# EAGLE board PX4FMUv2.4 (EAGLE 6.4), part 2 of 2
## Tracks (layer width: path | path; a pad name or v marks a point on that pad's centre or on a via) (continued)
GND  (via drill 0.2, 0.3) (continued)
  pour Top (isolate 0.254, rank 6, no thermals): 60.35,19.71 60.35,15.85 59.74,15.24 59.74,11.07 59.94,10.87 61.57,10.87 61.67,10.97 61.67,19.71 61.47,19.91 60.55,19.91
  pour Top (isolate 0.254, rank 6, no thermals): 51.71,35.36 59.03,35.26 59.13,35.15 59.13,28.85 59.03,28.75 51.71,28.85 51.51,29.06 51.61,35.26
  pour Top (isolate 0.254, rank 6, no thermals): 28.24,36.47 37.08,36.47 37.49,36.88 37.49,40.44 28.14,40.44 28.04,36.68
  pour Top (isolate 0.254, rank 6, no thermals): 52.22,17.88 57,17.88 57,13.31 52.22,13.31
  pour Top (isolate 0.254, rank 6, no thermals): 67.26,16.66 67.87,16.66 68.17,16.97 68.17,17.58 68.48,17.88 69.49,17.88 69.7,17.68 69.7,15.75 69.49,15.54 67.16,15.54 67.06,15.65 67.06,16.56 67.16,16.66
GPIO_EXT_1  (via drill 0.2)
  Top 0.152: v33.63,15.85 33.53,15.85 32.41,16.97 31.72,16.97 U101.8
  Vertical 0.152: v33.63,15.85 34.85,17.07 34.85,30.18 35.76,31.09 v38,31.09
  Bottom 0.152: J403.6 47.39,30.42 46.13,29.16 40.03,29.16 38.1,31.09 v38,31.09
GYRO_DRDY  (via drill 0.2)
  Top 0.152: U501.6 62.9,13.11 62.48,13.11 v61.98,12.6 | v43.48,12.29 43.48,12.5 42.8,13.18 U101.35 | U502.6 57.6,8.32 v57.81,8.33 | X503.5 57.13,4.6 v58.22,5.69
  Horizontal 0.152: v43.48,12.29 43.48,11.48 43.89,11.07 52.02,11.07 v52.22,11.28 | v53.14,5.69 v58.22,5.69
  Vertical 0.152: v58.22,5.69 58.22,8.13 58.01,8.33 v57.81,8.33 57.51,8.64 57.51,10.57 57.3,10.77 57.3,10.97 57.71,11.38 58.12,11.38 58.73,10.77 61.57,10.77 61.98,11.18 v61.98,12.6 | v52.22,11.28 52.22,6.6 v53.14,5.69
IO-!RESET  (via drill 0.2)
  Top 0.152: v19.51,16.66 19.51,16.71 U801.7 | U1002.3 13.66,7.26 v13.61,7.21 | v24.38,5.99 C801.P$2 23.77,4.77 23.77,3.09 S801.A1
  Horizontal 0.152: v13.61,7.21 14.94,8.53 v20.52,8.53
  Vertical 0.152: v20.52,8.53 20.52,15.65 v19.51,16.66
  Bottom 0.152: v24.38,5.99 22.86,5.99 20.52,8.33 v20.52,8.53
IO-!VDD_SERVO_IN_FAULT  (via drill 0.2)
  Top 0.152: U1001.4 12.46,4.74 v12.19,4.47 | v25.91,14.73 25.91,15.41 U801.38
  Horizontal 0.152: v12.19,4.47 12.39,4.27 15.65,4.27 16.46,5.08 16.46,7.21 17.27,8.03 20.73,8.03 21.03,8.33 22.15,8.33 25.7,11.89 25.7,13.51 25.6,13.61 25.6,14.43 v25.91,14.73
IO-BOOT0  (via drill 0.2)
  Top 0.152: U801.44 25.26,19.01 | 25.26,19.01 R801.P$1 | 25.26,19.01 25.26,19.14 23.67,20.73 v23.16,20.73
  Bottom 0.152: v23.16,20.73 23.57,20.73 IO-BOOT1101.P$1
IO-BOOT1
  Top 0.152: R802.P$1 17.92,9.54 U801.20
IO-CH1
  Top 0.152: U801.10 17.03,17.07 15.85,17.07 15.57,16.79 U902.9
IO-CH1-PROT
  Top 0.406: J901.28 8.33,21.97 8.33,19.21 R917.P$2
IO-CH2
  Top 0.152: U801.11 16.73,16.66 16.26,16.66 15.88,16.29 U902.8
IO-CH3
  Top 0.152: U902.7 16.22,15.79 16.87,15.14 22.05,15.14 23.57,16.66 23.57,18.02 U801.45
IO-CH4  (via drill 0.2)
  Top 0.152: U902.6 15.5,15.29 v15.54,15.24 | v22.96,18.12 U801.46
  Horizontal 0.152: v22.96,18.12 22.49,18.12 19.61,15.24 v15.54,15.24
IO-CH5
  Top 0.152: U902.5 15.49,14.79 16.05,14.22 16.05,11.68 16.26,11.48 17.03,11.48 U801.16
IO-CH6
  Top 0.152: U902.4 15.38,14.29 15.75,13.92 15.75,11.48 16.05,11.18 17.43,11.18 U801.17
IO-CH7
  Top 0.152: U902.3 15.27,13.79 15.44,13.61 15.44,11.28 15.85,10.87 17.83,10.87 U801.18
IO-CH8
  Top 0.152: U801.19 18.23,10.57 15.65,10.57 15.14,11.07 15.14,12.09 15.04,12.19 14.02,12.19 13.76,12.46 U902.1
IO-CH8-PROT
  Top 0.152: 8.44,10.47 R905.P$2
  Top 0.406: J901.7 7.72,7.64 7.72,9.75 8.44,10.47
IO-SWCLK  (via drill 0.2)
  Top 0.152: U801.37 26.44,15.24 v26.42,15.24
  Bottom 0.152: JX802.4 16.1,18.85 17.37,17.58 23.06,17.58 25.4,15.24 v26.42,15.24
IO-SWDIO  (via drill 0.2)
  Top 0.152: v25.09,14.02 25.09,13.96 U801.34
  Bottom 0.152: JX802.2 15.75,17.58 16.15,17.17 22.66,17.17 25.09,14.73 v25.09,14.02
IO-SWO  (via drill 0.2)
  Top 0.152: U801.39 25.74,15.95 v25.7,15.95
  Bottom 0.152: JX802.6 22.15,20.12 25.7,16.56 v25.7,15.95
IO-USART1_RX  (via drill 0.2)
  Top 0.152: U801.31 v24.69,12.24
  Horizontal 0.152: v24.69,12.24 24.13,12.8 15.44,12.8 14.83,13.41 v13.01,13.41 | v11.68,0.61 18.95,0.61 v19.1,0.46
  Vertical 0.152: v15.75,27.13 13.01,24.38 v13.01,13.41 13.01,10.16 11.38,8.53 11.38,2.85 11.68,2.54 v11.68,0.61
  Bottom 0.152: J801.P$3 15.93,27.31 v15.75,27.13 | v19.1,0.46 19.25,0.61 19.71,0.61 JX801.2
IO-USART1_TX  (via drill 0.2)
  Top 0.152: v24.08,23.06 24.18,23.16 R101.P$2 | v24.08,12.19 24.08,12.14 U801.30
  Vertical 0.152: v24.08,23.06 v24.08,12.19 23.27,12.19 22.86,11.79 22.86,11.18 23.27,10.77 23.27,3.45 22.25,2.44 v22.15,2.44
  Bottom 0.152: JX801.1 22.86,2.13 22.55,2.44 v22.15,2.44
IO-VDD_3V3  (via drill 0.2, 0.3)
  Top 0.254: U801.48 22.45,20.49 C803.P$1 22.45,21.45 v22.35,21.54 21.95,21.95 D701.C | C804.P$1 27.32,14.13 v27.23,14.22 27.23,13.55 U801.36 | v11.28,12.8 11.26,12.82 U902.19 | v14.73,12.7 14.73,13.26 U902.2 | v13.82,16.26 13.76,16.32 U902.10 13.94,17.48 14.22,17.48 | U801.9 17.33,17.48 14.22,17.48 | C802.P$1 21.45,9.25 v21.54,9.35 21.38,9.5 U801.24 | C903.P$1 14.32,17.57 14.22,17.48 | U903.8 13.15,3.72 C901.P$1 12.61,3.76 v12.29,3.76
  Bottom 0.406: J702.1 22.32,21.57 v22.35,21.54 | JX802.1 11.48,17.58 v12.19,18.29
  other vias: 11.07,10.36 11.58,10.36
  pour Power: 7.72,23.98 7.72,0 28.04,0 28.04,16.66 20.73,23.98
  pour Top (isolate 0.254, rank 3, no thermals): 13.31,9.14 13.31,10.36 13.21,10.46 12.29,10.46 11.89,10.87 11.89,11.58 11.79,11.68 10.97,11.68 10.87,11.58 10.87,9.55 10.97,9.45 11.89,9.45 12.29,9.86 12.9,9.86 13,9.75 13,9.14 13.11,9.04 13.21,9.04
IO-VDD_5V5  (via drill 0.3)
  Top 0.25: v14.22,3.05 14.53,3.05 C1005.P$1
  Top 0.305: v14.58,7.32 U1002.4 | v12.09,7.73 U1002.1
  Top 0.406: C1001.P$1 v14.58,7.32 | v12.09,7.73 11.67,7.32 D1001.3
  Vertical 0.406: v14.22,3.05 14.22,6.96 v14.58,7.32
  Power 0.406: J901.2 5.05,2.44 7.52,2.44 8.53,3.45 10.57,3.45 10.97,3.05 v14.22,3.05
  Bottom 0.254: LED702.A 8.8,3.45 10.46,3.45 10.93,2.98 LED703.A 14.16,2.98 v14.22,3.05 14.29,2.98 LED705.A 16.42,2.98
  Bottom 0.406: v12.09,7.73 13.02,7.73 13.11,7.82 14.07,7.82 v14.58,7.32
MAG_DRDY  (via drill 0.2)
  Top 0.152: U504.9 63.08,4.86 v62.99,4.78 | v58.12,4.78 57.63,4.29 X503.4 | U101.36 44.09,12.61 v44.09,12.09
  Horizontal 0.152: v62.99,4.78 v58.12,4.78 57.61,4.27 57.61,2.85 57,2.23 49.17,2.23 47.24,4.17 v43.69,4.17
  Vertical 0.152: v43.69,4.17 43.69,11.68 v44.09,12.09
MPU_DRDY  (via drill 0.2)
  Top 0.152: U505.12 63.27,18.05 63.09,17.88 63.09,16.76 v62.59,16.26 | U101.62 44.91,25.91 v46.43,25.91
  Horizontal 0.152: v62.59,16.26 62.38,16.26 60.76,17.88 47.75,17.88 46.74,18.9 46.74,19.71 v46.43,20.02
  Vertical 0.152: v46.43,20.02 46.43,20.12 46.53,20.22 46.53,25.81 v46.43,25.91
N$1
  Top 0.152: U101.13 31.9,13.61 31.9,12.7 32.26,12.34 | 32.26,12.34 C103.P$2 | X101.1 30.67,10.76 32.26,12.34
N$2
  Top 0.152: U101.12 31.24,13.66 C102.P$1 31.24,12.14 29.46,10.36 27.92,10.36 X101.3
N$3
  Top 0.152: R922.P$1 11.88,19.71 R918.P$2
N$4  (via drill 0.2, 0.3)
  Top 0.25: U1001.8 15.4,6.34 v15.54,6.2
  Top 0.254: v9.55,6.71 9.21,6.37 D1001.2
  Power 0.406: v9.55,6.71 9.86,7.01 12.29,7.01 13.11,7.82 14.12,7.82 14.33,8.03 14.83,8.03 15.54,7.32 v15.54,6.2
N$5  (via drill 0.3)
  Top 0.254: v34.04,37.59 D201.C
  Top 0.406: L201.P$2 v34.04,37.59 v33.43,37.59
  Bottom 0.406: J201.1 34.04,36.97 v34.04,37.59 v33.43,37.59
N$6
  Top 0.152: U504.15 65.13,1.32 64.92,1.12 C509.P$1
N$7  (via drill 0.2)
  Top 0.152: v8.33,39.93 8.85,39.41 R711.P$2
  Bottom 0.152: LED704.C v8.33,39.93
N$8
  Top 0.152: U101.73 41.06,29.85 C613.P$1
N$9  (via drill 0.15, 0.2)
  Top 0.152: R712.P$2 v24.28,6.6
  Horizontal 0.152: v24.28,6.6 23.88,6.6 23.27,5.99 23.27,2.23 22.55,1.52 17.07,1.52 v16.46,2.13
  Bottom 0.152: v16.46,2.13 LED705.C
N$10
  Top 0.152: U504.2 67.78,3.36 C510.P$1
N$11
  Top 0.15: C602.P$2 57.51,11.18 58.32,11.99 58.32,13.51 57.96,13.87 U603.6
N$12
  Top 0.152: U101.49 47.14,18.75 47.14,19.1 47.95,19.91 49.44,19.91 C611.P$1
N$13
  Top 0.152: R707.P$2 R3.P$1
N$14  (via drill 0.2)
  Top 0.152: R215.P$2 28.35,25.09 v27.94,25.5
  Horizontal 0.152: v35.36,7.82 35.36,8.23 32.31,11.28 v26.72,11.28
  Vertical 0.152: v26.72,11.28 26.72,12.7 27.74,13.72 27.74,19.61 26.52,20.83 26.52,24.08 v27.94,25.5
  Bottom 0.152: J203.4 34.83,6.28 35.36,6.81 v35.36,7.82
N$15  (via drill 0.2)
  Top 0.152: U801.12 17.24,15.44 21.54,15.44 v22.55,16.46 | v23.47,22.86 23.06,23.27 R803.P$1
  Vertical 0.152: v22.55,16.46 23.67,17.58 23.67,22.66 v23.47,22.86
N$16  (via drill 0.2)
  Top 0.152: U801.13 17.07,13.64 17.07,14.22 17.68,14.83 22.55,14.83 v24.59,16.87 | v25.3,23.06 R804.P$1
  Vertical 0.152: v24.59,16.87 25.3,17.58 v25.3,23.06
N$17
  Top 0.152: U504.3 67.16,3.86 67.67,4.37 68.57,4.37 C510.P$2
N$18
  Top 0.152: U801.6 17.98,18.95 C806.P$2 16.51,20.16 X801.1
N$19  (via drill 0.2)
  Top 0.152: R216.P$2 49.48,23.77 v49.68,23.98
  Horizontal 0.152: v35.76,25.6 37.19,25.6 37.9,24.89 40.03,24.89 40.23,24.69 41.45,24.69 41.96,25.2 48.36,25.2 v49.68,23.98
  Vertical 0.152: v35.36,4.57 35.97,5.18 35.97,25.4 v35.76,25.6
  Bottom 0.152: v35.36,4.57 34.9,5.03 J203.5
N$20
  Top 0.152: U1001.7 14.79,5.84 R1001.P$2
N$21
  Top 0.254: R608.P$2 22.56,31.46 D2.C
N$22
  Top 0.152: U801.5 18.44,19.19 C805.P$1 16.64,21.47 X801.3
N$23  (via drill 0.2)
  Top 0.152: U101.69 41.07,27.03 40.74,27.03 v40.23,27.53 | v24.18,25.5 R101.P$1
  Bottom 0.152: v40.23,27.53 40.23,28.45 38.2,30.48 37.49,30.48 37.29,30.68 35.97,30.68 32.31,27.03 25.7,27.03 v24.18,25.5
N$24  (via drill 0.2)
  Top 0.152: R706.P$1 8.85,30.28 | 8.85,30.28 R705.P$2 | U702.2 14.1,27.64 v13.01,27.64 | v10.36,30.28 8.85,30.28
  Horizontal 0.152: v13.01,27.64 v10.36,30.28
N$25
  Top 0.152: U702.8 10.01,27.07 R702.P$1 8.85,26.23 R703.P$2
N$26  (via drill 0.2)
  Top 0.152: v14.43,39.93 14.94,39.41 R3.P$2
  Bottom 0.152: LED701.C 13.27,39.93 v14.43,39.93
N$27  (via drill 0.2)
  Top 0.152: U702.1 14.06,27.07 13.61,26.62 10.46,26.62 R703.P$1 9.85,25.4 | C703.P$1 9.85,25.4 | v9.35,25.4 9.85,25.4
  Bottom 0.152: J701.1 15.15,16.27 14.66,16.76 8.53,16.76 7.72,17.58 7.72,23.57 9.35,25.2 v9.35,25.4
N$28
  Top 0.152: R701.P$1 10.58,27.72 U702.7
N$29  (via drill 0.2)
  Top 0.152: R708.P$2 20.94,0.81 21.44,0.81 v21.54,0.71
  Horizontal 0.152: v10.77,1.12 11.89,1.12 12.09,0.91 21.34,0.91 v21.54,0.71
  Bottom 0.152: LED702.C 10.4,1.49 v10.77,1.12
N$30
  Top 0.152: U502.14 C505.P$1
N$31
  Top 0.406: R914.P$2 8.13,11.79 7.72,11.38 7.72,10.67 6.3,9.25 J901.10
N$32
  Top 0.152: U702.5 11.83,31.74 12.23,32.14 L701.P$2
N$33  (via drill 0.2)
  Top 0.152: R404.P$2 v47.95,2.03
  Bottom 0.152: v47.95,2.03 51.51,2.03 55.79,6.32 J401.2
N$34
  Top 0.152: R616.P$1 60.5,26.17 U602.7
N$35
  Top 0.152: U501.14 68.06,12.48 C504.P$1
N$36
  Top 0.152: U702.6 11.75,28.45 10.97,28.45 9.85,29.57 R705.P$1 10.97,29.67 11.07,29.77 C704.P$1
N$37  (via drill 0.2)
  Top 0.152: v48.36,1.52 47.75,0.91 R405.P$2
  Bottom 0.152: J401.3 55.05,5.07 51.51,1.52 v48.36,1.52
N$38  (via drill 0.2)
  Top 0.152: D902.C v9.96,5.18 R910.P$1 | v16.15,8.03 16.36,8.23 R901.P$2 | U903.3 10.24,1.4 10.57,1.73 v10.97,1.73
  Horizontal 0.152: v9.96,5.18 12.5,5.18 13.01,4.57 15.34,4.57 16.05,5.28 16.05,7.92 v16.15,8.03
  Vertical 0.152: v9.96,5.18 10.67,4.47 10.67,2.03 v10.97,1.73
N$39  (via drill 0.2)
  Top 0.152: R709.P$2 22.45,3.67 v22.45,3.45 | v17.98,3.05 R4.P$1
  Horizontal 0.152: v22.45,3.45 21.13,2.13 18.59,2.13 17.98,2.74 v17.98,3.05
N$40  (via drill 0.15)
  Top 0.152: R4.P$2 16.86,1.13 v15.85,2.13
  Bottom 0.152: LED703.C 12.43,1.52 15.24,1.52 v15.85,2.13
N$41  (via drill 0.2)
  Top 0.4: D402.C v53.44,36.37 L402.P$2
  Bottom 0.4: 55.47,36.37 v53.44,36.37
  Bottom 0.406: 55.47,36.37 55.77,36.67 J403.1
N$42  (via drill 0.3)
  Top 0.254: D401.C 62.49,3.44 L401.P$2
  Top 0.406: L401.P$2 v61.37,6.5
  Bottom 0.254: J402.1 64.5,6.5
  Bottom 0.406: 64.5,6.5 v61.37,6.5 60.3,7.57 J401.1
N$43
  Top 0.15: 12.26,12.46 12.09,12.29 10.77,12.29 10.26,11.79 10.26,10.77 10.06,10.57 R905.P$1
  Top 0.152: U902.20 12.26,12.46
N$44
  Top 0.152: U902.18 11.22,13.82 10.57,13.82 10.57,12.91 R914.P$1
N$45
  Top 0.152: U902.17 10.22,14.29 10.16,14.22 10.16,13.41 9.75,13.01 R906.P$1
N$46  (via drill 0.3)
  Top 0.61: D1001.1 8.65,8.21 v8.64,7.62 | v12.19,24.08 12.19,25.38 F1001.2
  Power 0.61: v8.64,7.62 8.64,17.68 12.19,21.23 v12.19,24.08
N$47
  Top 0.152: R1105.P$2 57.19,36.27 R1106.P$1 C1108.P$1 58.33,36.27 59.44,36.27 59.97,35.73 U1101.P$1
N$48  (via drill 0.3)
  Top 0.254: D404.C 37.09,8.12 L403.P$2 | 39,8.12 v39.01,8.13
  Top 0.406: L403.P$2 39,8.12
  Bottom 0.254: J405.1 41.62,7.42
  Bottom 0.406: v39.01,8.13 39.58,7.57 39.73,7.42 41.62,7.42
N$49
  Top 0.152: U902.16 10,14.79 R915.P$1
N$50
  Top 0.152: U505.10 62.5,19.05 C512.P$1
N$51
  Top 0.2: U505.20 68.99,18.55 C515.P$1
N$53
  Top 0.152: U902.15 9.6,15.29 R907.P$1
N$54
  Top 0.152: R1107.P$1 57.09,35.15 R1106.P$2 57.2,35.66 57.3,35.76 59.33,35.76 59.54,35.56 59.54,35.05 59.33,34.85 59.33,34.34 59.6,34.08 U1101.P$2
N$55
  Top 0.152: R1109.P$2 57.19,33.73 R1110.P$1 C1109.P$1 58.63,33.72 58.83,33.53 59.93,33.53 U1101.P$3
N$56
  Top 0.152: R1111.P$1 57.09,32.61 R1110.P$2 57.2,33.12 57.3,33.22 58.93,33.22 59.08,33.08 U1101.P$4
N$57  (via drill 0.2)
  Top 0.152: v22.45,7.11 22.46,7.11 R710.P$1
  Bottom 0.152: J702.2 25.3,20.32 24.79,19.81 24.79,18.29 26.92,16.15 26.92,14.94 26.62,14.63 26.62,12.8 22.45,8.64 v22.45,7.11
N$58
  Top 0.152: U902.14 10.32,15.79 R916.P$1
N$59
  Top 0.152: U902.13 10.54,16.29 10.16,16.66 10.16,17.16 R908.P$1
N$60
  Top 0.152: U902.12 11.26,17.6 9.75,19.1 R917.P$1
N$61
  Top 0.152: R902.P$1 10.56,32.82 12.09,32.82 12.66,33.39 U901.20
N$62
  Top 0.152: R911.P$1 11.04,34.51 U901.18
N$63
  Top 0.152: R903.P$1 10.32,35.01 U901.17
N$64
  Top 0.152: R912.P$1 10.1,35.51 U901.16
N$65
  Top 0.152: R904.P$1 10.82,36.01 U901.15
N$66
  Top 0.152: U901.14 11.04,36.51 10.57,36.98 10.57,37.48 R913.P$1
N$67
  Top 0.152: R1114.P$1 R1113.P$2 57.2,30.48 57.3,30.58 58.83,30.58 59.33,31.09 59.33,31.8 59.61,32.08 U1101.P$6
N$68
  Top 0.152: R911.P$2 8.85,33.23
  Top 0.305: 8.85,33.23 7.62,32 7.62,30.68 6.3,29.36
  Top 0.406: J901.34 6.3,29.36
N$69
  Top 0.152: R1112.P$2 57.09,31.19 R1113.P$1 C1110.P$1 58.83,31.09 59.03,31.29 59.03,32.31 59.3,32.58 U1101.P$5
N$70
  Top 0.152: R201.P$1 26.01,30.89 26.07,30.82 U201.20
N$71
  Top 0.406: J901.13 8,13.01 R906.P$2
N$72
  Top 0.406: J901.16 6.68,14.22 R915.P$2
N$73
  Top 0.406: J901.19 7.5,16.38 R907.P$2
N$74
  Top 0.406: J901.22 6.3,18.8 R916.P$2
N$75
  Top 0.406: J901.25 7.39,21.46 7.72,21.13 7.72,18.6 R908.P$2
N$77
  Top 0.406: R903.P$2 8.33,34.54 7.82,34.04 7.82,33.15 J901.37
N$78
  Top 0.406: R912.P$2 7.9,35.76 J901.40
N$79
  Top 0.406: J901.43 8.57,36.7 R904.P$2
N$80
  pour Top (isolate 0.254, rank 6, no thermals): 56.59,21.74 57.61,21.74 57.61,19.1 56.59,19.1
N$81
  Top 0.152: Q601.B 56.15,19.74 R620.P$1
N$82
  Top 0.152: U201.18 27.6,32.54 27.03,33.12 R208.P$1
N$83
  Top 0.152: U201.17 28.1,32.86 R202.P$1
N$84
  Top 0.152: U201.16 28.6,33.48 R209.P$1
N$85
  Top 0.152: U201.15 29.1,35.29 R203.P$1
N$86
  Top 0.152: U201.14 29.6,34.58 R210.P$1
N$87
  Top 0.152: U201.13 30.1,33.86 R204.P$1
N$88
  Top 0.152: U201.12 30.6,33.14 R211.P$1
N$89
  Top 0.152: U202.13 30.76,4.5 R207.P$1
N$90
  Top 0.152: R214.P$1 31.89,5 U202.12
N$91
  Top 0.152: R205.P$1 27.23,5.28 30.01,2.5 U202.17
N$92
  Top 0.152: U202.16 30.02,3 27.53,5.49 27.53,6.2 27.23,6.5 R212.P$1
N$93
  Top 0.152: U202.15 30.03,3.5 27.84,5.69 27.84,6.8 R206.P$1
N$94
  Top 0.152: U202.14 30.04,4 28.14,5.89 28.14,7.72 28.04,7.82 R213.P$1
N$95
  Top 0.152: R704.P$2 49.17,12.19 48.77,12.6 48.58,12.79 U701.6
N$96
  Top 0.152: U601.7 37.44,38.45 R617.P$1
N$97
  Top 0.3: U1101.P$18 64.04,34.58 64.31,34.85 64.31,38.1 64.8,38.58 U1102.P$1
  Top 0.4: 66.14,38.58 66.14,39.63 C1105.P$1
  Top 0.406: U1102.P$1 66.14,38.58 66.14,37.26 U1102.P$3
N$98  (via drill 0.3)
  Top 0.254: D403.C 46.22,14.62 L404.P$2
  Top 0.406: L404.P$2 v47.14,15.34
  Bottom 0.406: v47.14,15.34 47.14,22.76 46.02,23.88 44.5,23.88 43.28,22.66 41.94,22.66 J404.1
N$99
  Top 0.406: J901.4 7.8,5.18 R910.P$2
N$100  (via drill 0.3)
  Top 0.254: D203.C 33.49,8.07 L203.P$2 32.51,9.06 v32.51,9.96
  Bottom 0.254: 32.44,10.03 v32.51,9.96
  Bottom 0.406: v32.51,9.96 32.59,10.03 J203.1 | J204.1 32.44,10.03
N$101  (via drill 0.3)
  Top 0.254: D202.C 24.78,34.24 | L202.P$2
  Top 0.406: 24.78,34.24 L202.P$2 | L202.P$2 v24.79,36.17
  Bottom 0.254: 26.15,36.98 J202.1
  Bottom 0.406: J202.1 25.48,36.86 v24.79,36.17
N$102
  Top 0.152: L1102.P$2 61.06,29.77 60.76,29.46 R1102.P$2
N$103
  Top 0.152: L1101.P$2 R1101.P$2
N$104
  Top 0.152: U1002.6 13.66,9.81 C1002.P$1
N$105
  Top 0.15: R1115.P$2 60.05,36.26 60.62,35.69 U1101.P$24
N$106
  Top 0.254: 66.14,32.99 66.14,33.02
  Top 0.3: U1101.P$16 64.26,33.58 65,34.31 U1103.P$1
  Top 0.4: U1103.P$1 66.14,34.31 | 66.14,34.31 66.14,33.02 | U1103.P$3 66.14,32.99 | 66.14,34.31 66.14,35.37 C1106.P$1
N$107
  Top 0.254: 66.14,28.73 66.14,28.75
  Top 0.3: U1101.P$14 64.45,32.58 64.62,32.41 64.62,30.38 64.95,30.05 U1104.P$1
  Top 0.4: 66.14,30.05 66.14,31.1 C1107.P$1
  Top 0.406: U1104.P$1 66.14,30.05 66.14,28.75 | U1104.P$3 66.14,28.73
N$109
  Top 0.152: U1104.P$4 64.92,28.07 64.92,29.36 | 64.92,29.36 65.46,29.36 U1104.P$2 | U1101.P$13 63.77,30.51 64.92,29.36
N$110
  Top 0.254: 9.96,22.27 D903.C
  Top 0.406: D1.CATHODE 9.96,22.27 | D903.C 9.77,22.65 L901.P$1
N$113
  Top 0.152: U1101.P$15 64.37,33.08 64.47,33.17 | 64.47,33.17 64.95,33.66 U1103.P$2 | U1103.P$4 65.1,32.33 65.02,32.41 65.02,32.61 64.47,33.17
N$115
  Top 0.152: U1102.P$2 64.95,37.92 64.72,37.69 64.72,36.58 | U1101.P$17 64.15,34.08 64.72,34.65 64.72,36.58 | U1102.P$4 64.75,36.6 64.72,36.58
OTG_DM1  (via drill 0.2)
  Top 0.152: U302.1 44.39,33.42 44.5,33.53 44.5,34.34 v44.3,34.54 | 44.39,34.45 v44.3,34.54 | J301.D- 44.13,34.71 v44.3,34.54
  Bottom 0.152: v44.3,34.54 43.79,34.54 43.37,34.12 J302.3
OTG_DP1  (via drill 0.2)
  Top 0.152: J301.D+ v43.48,34.95 | U302.3 43.39,33.42 43.28,33.53 43.28,34.75 v43.48,34.95 | v43.48,34.95 43.39,34.86 v43.48,34.95
  Bottom 0.152: J302.2 43.06,35.37 v43.48,34.95
OTG_FS_DM
  Top 0.152: U101.70 44.39,31.05 U302.6
OTG_FS_DP
  Top 0.152: U101.71 43.39,30.76 U302.4
PB2-BOOT1
  Top 0.152: U101.37 44.76,12.65 R102.P$1
PPM-SBUS-PROT
  Top 0.406: J901.1 7.72,2.56 7.72,3.66 8.13,4.06 R909.P$2
PPM_INPUT  (via drill 0.2)
  Top 0.152: R909.P$1 v9.96,4.06 D901.C 10.47,3.55 11.18,2.85 v11.18,2.34 10.57,2.34 10.28,2.05 U903.2 | U801.29 23.98,11.54 v23.98,11.58
  Horizontal 0.152: v24.99,3.35 24.99,3.15 23.06,1.22 12.29,1.22 v11.18,2.34
  Vertical 0.152: v24.99,3.35 23.77,4.57 23.77,10.87 23.98,11.07 v23.98,11.58
PRESSURE_SENS  (via drill 0.2)
  Top 0.152: R403.P$2 69.59,8.95 69.7,8.84 69.7,7.01 69.6,6.91 C401.P$1 R406.P$1 68.18,5.88 v68.17,5.89 | U101.34 41.57,13.72 v41.55,13.72
  Horizontal 0.152: v40.23,8.23 40.54,7.92 57.2,7.92 57.71,7.42 61.27,7.42 62.79,5.89 v68.17,5.89
  Vertical 0.152: v41.55,13.72 40.64,12.8 40.64,8.94 40.23,8.53 v40.23,8.23
PRESSURE_SENS_IN  (via drill 0.2)
  Top 0.152: R406.P$2 68.18,4.88 v68.17,4.88
  Bottom 0.152: ADC_PR.P$1 J402.2 67.77,5.28 v68.17,4.88
RGB_LED_3  (via drill 0.2)
  Top 0.152: U701.9 50.08,13.61 v50.39,13.92
  Bottom 0.152: v50.39,13.92 51.71,13.92 52.93,15.34 52.93,16.36 52.73,16.56 52.73,18.83 U703.C1
  pour Bottom (isolate 0.254, rank 2, no thermals): 52.43,19.81 52.43,14.83 56.18,14.83 56.18,19.81
RGB_LED_4  (via drill 0.2)
  Top 0.152: U701.8 v49.58,13.82
  Bottom 0.152: v49.58,13.82 49.58,13.92 51.61,15.95 U703.C2
  pour Bottom (no thermals): 51.31,19.81 51.31,14.83 51.92,14.83 51.92,19.81
RGB_LED_14  (via drill 0.2)
  Top 0.152: U701.7 49.08,14.23 v49.58,14.73
  Bottom 0.152: U703.C3 50.51,16.44 49.58,15.51 v49.58,14.73
  pour Bottom (no thermals): 50.8,19.81 50.8,14.83 47.14,14.83 47.14,19.81
RSSI_IN  (via drill 0.2)
  Top 0.152: R901.P$1 v16.36,10.06 | v16.87,12.09 16.93,12.09 U801.15 | v25.2,13.11 25.24,13.11 U801.33
  Horizontal 0.152: v16.36,10.06 16.46,9.96 23.27,9.96 25.2,11.89 v25.2,13.11
  Vertical 0.152: v16.36,10.06 16.36,11.58 v16.87,12.09
SAFETY  (via drill 0.2)
  Top 0.152: U801.41 26.21,17.84 v26.21,17.88 27.23,18.9 R713.P$1
  Bottom 0.152: J702.3 26.33,18 v26.21,17.88
SBUS_INPUT  (via drill 0.15, 0.2)
  Top 0.152: U903.6 13.9,1.4 14.33,1.83 v14.33,2.34 | U801.22 18.59,8.8 v18.59,7.52
  Horizontal 0.15: v16.87,4.47 16.87,2.95 16.56,2.64 14.63,2.64 v14.33,2.34
  Horizontal 0.152: v16.87,4.47 16.87,5.79 v18.59,7.52
SBUS_OUTPUT
  Top 0.152: U903.5 13.86,0.75 14.83,1.73 14.83,2.34 15.44,2.95 16.66,2.95 16.87,3.15 16.87,3.76 17.37,4.27 17.37,6.2 18.09,6.91 18.09,9 U801.21
SDIO_CK  (via drill 0.2)
  Top 0.152: v36.88,26.92 36.85,26.92 U101.80
  Bottom 0.152: v36.88,26.92 36.98,27.03 40.64,27.03 40.95,27.33 55.58,27.33 61.65,21.26 U301.5
SDIO_CMD  (via drill 0.2)
  Top 0.152: R303.P$1 33.73,29.37 33.73,27.92 U101.83 35.34,26.31 v35.36,26.31
  Bottom 0.152: v35.36,26.31 37.08,26.31 37.49,26.72 40.95,26.72 41.25,27.03 41.35,27.03 55.37,27.03 63.34,19.06 U301.3
SDIO_D0  (via drill 0.2)
  Top 0.152: U101.65 44.2,27.33 44.5,27.33 R304.P$1 46.18,27.89 v46.23,27.94
  Bottom 0.152: v46.23,27.94 46.63,28.35 55.07,28.35 59.74,23.67 63.4,23.67 63.62,23.46 U301.7
SDIO_D1  (via drill 0.2)
  Top 0.152: U101.66 44.01,27.84 v44.2,27.84 44.2,28.65 R305.P$1
  Bottom 0.152: v44.2,27.84 45.01,28.65 55.27,28.65 59.33,24.59 59.37,24.56 59.94,23.98 62.79,23.98 63.37,24.56 U301.8
SDIO_D2  (via drill 0.2)
  Top 0.152: R301.P$1 35.71,30.43 35.36,30.07 35.36,29.83 U101.78 38.3,26.88 v38.3,25.91
  Bottom 0.152: v38.3,25.91 38.51,26.11 41.66,26.11 41.96,26.42 54.97,26.42 63.4,17.98 63.4,17.27 63.81,16.86 U301.1
SDIO_D3  (via drill 0.2)
  Top 0.152: R302.P$1 34.9,29.58 U101.79 37.69,26.79 v37.69,26.21
  Bottom 0.152: v37.69,26.21 37.9,26.42 41.35,26.42 41.66,26.72 55.17,26.72 63.93,17.96 U301.2
SERIAL1_CTS  (via drill 0.2)
  Top 0.152: v32.92,33.12 32.72,33.33 R211.P$2
  Bottom 0.152: J201.4 arc90 34.13,33.12 v32.92,33.12
SERIAL1_RTS  (via drill 0.2)
  Top 0.152: v32.82,33.83 32.11,34.54 R204.P$2
  Bottom 0.152: J201.5 32.76,31.86 32.11,32.51 32.11,33.12 v32.82,33.83
SERIAL1_RX  (via drill 0.2)
  Top 0.152: R203.P$2 31.29,36.48 31.29,35.36 31.5,35.15 32.51,35.15 32.92,34.75 v32.92,34.44
  Bottom 0.152: J201.3 33,34.36 v32.92,34.44 32,34.44 S1RX.P$1
SERIAL1_TX  (via drill 0.2)
  Top 0.152: R210.P$2 32.41,35.76 v32.72,36.07
  Bottom 0.152: J201.2 33.17,35.61 v32.72,36.07 v32.72,38.2 32.72,38.71 32.21,39.22 S1TX.P$1
SERIAL2_CTS  (via drill 0.2)
  Top 0.152: R208.P$2 v24.49,33.12
  Bottom 0.152: J202.4 26.26,33.12 v24.49,33.12
SERIAL2_RTS  (via drill 0.2)
  Top 0.152: R201.P$2 v24.59,30.18
  Bottom 0.152: J202.5 24.85,31.86 24.59,31.6 v24.59,30.18
SERIAL2_RX  (via drill 0.2)
  Top 0.152: R202.P$2 27.74,35.04 v27.74,35.36
  Bottom 0.152: S2RX.P$1 24.89,34.14 25.09,34.34 26.25,34.34 J202.3 27.45,34.36 27.74,34.65 v27.74,35.36
SERIAL2_TX  (via drill 0.2)
  Top 0.152: R209.P$2 v28.45,35.36
  Bottom 0.152: J202.2 27.28,35.61 27.53,35.87 27.94,35.87 v28.45,35.36 30.38,35.36 S2TX.P$1
SERIAL3_RX  (via drill 0.2)
  Top 0.152: R207.P$2 v30.48,6.4
  Bottom 0.152: S3RX.P$1 30.48,4.88 v30.48,6.4 31.9,6.4 33.03,7.53 J203.3
SERIAL3_TX  (via drill 0.2)
  Top 0.152: R214.P$2 v31.7,6.91
  Bottom 0.152: S3TX.P$1 35.36,10.57 35.36,9.04 35.1,8.78 J203.2 32.97,8.78 32.72,8.53 32.72,7.92 v31.7,6.91
SERIAL4_RX  (via drill 0.2)
  Top 0.152: R206.P$2 25.3,7.72 v25.09,7.52
  Bottom 0.152: J204.3 25.11,7.53 v25.09,7.52 S4RX.P$1
SERIAL4_TX  (via drill 0.2)
  Top 0.152: R213.P$2 25.2,8.94 v25.09,8.84
  Bottom 0.152: J204.2 26.27,8.84 v25.09,8.84 24.59,9.35 S4TX.P$1
SERIAL5_RX  (via drill 0.2)
  Top 0.152: R205.P$2 25.2,5.28 v25.09,5.18
  Bottom 0.152: J204.5 25.24,5.03 v25.09,5.18 25.09,4.47 24.38,3.76 S5_RX.P$1
SERIAL5_TX  (via drill 0.2)
  Top 0.152: R212.P$2 25.3,6.5 v25.09,6.3
  Bottom 0.152: J204.4 26.31,6.3 v25.09,6.3 24.89,6.1 24.89,5.69 S5_TX.P$1
SERIAL_FMU_TO_IO  (via drill 0.2)
  Top 0.152: v25.3,25.5 R804.P$2 | U101.63 43.28,24.99 42.88,24.99 v40.44,22.55
  Horizontal 0.152: v25.3,25.5 26.82,27.03 31.5,27.03 36.37,22.15 40.03,22.15 v40.44,22.55
SERIAL_IO_TO_FMU  (via drill 0.2)
  Top 0.152: v23.67,26.01 23.06,25.4 R803.P$2 | U101.64 42.88,25.3 42.37,25.3 v39.73,22.66
  Horizontal 0.152: v23.67,26.01 25.3,26.01 26.62,27.33 31.7,27.33 36.37,22.66 v39.73,22.66
SPI_EXT_MISO  (via drill 0.2)
  Top 0.152: U101.4 30.79,18.86 v30.79,18.9
  Horizontal 0.152: v53.65,32.21 52.93,31.5 43.38,31.5 42.06,32.82 v36.27,32.82
  Vertical 0.152: v36.27,32.82 36.17,32.82 34.24,30.89 34.24,23.16 30.89,19.81 30.89,19 v30.79,18.9
  Bottom 0.152: J403.3 55.61,34.17 v53.65,32.21
SPI_EXT_MOSI  (via drill 0.2)
  Top 0.152: U101.5 31.39,18.76 v31.39,19.1
  Horizontal 0.152: v54.56,32.21 54.15,31.8 53.95,31.8 53.34,31.19 43.18,31.19 42.06,32.31 v36.68,32.31
  Vertical 0.152: v36.68,32.31 36.37,32.31 34.54,30.48 34.54,22.96 31.39,19.81 v31.39,19.1
  Bottom 0.152: J403.4 55.27,32.92 v54.56,32.21
SPI_EXT_SCK  (via drill 0.2)
  Top 0.152: U101.1 29.51,19.71 v29.77,19.71
  Horizontal 0.152: v53.54,32.92 53.14,32.51 43.38,32.51 42.06,33.83 v36.37,33.83
  Vertical 0.152: v36.37,33.83 35.66,33.83 33.63,31.8 33.63,23.57 v29.77,19.71
  Bottom 0.152: J403.2 56.04,35.42 v53.54,32.92
SPI_INT_MISO  (via drill 0.15, 0.2)
  Top 0.152: 63.91,14.64 U501.4 63.91,14.76 v63.91,15.44 | v42.27,10.87 42.27,10.9 U101.31 | U505.9 64.26,19.55 64.52,19.81 64.52,20.32 64.82,20.62 66.45,20.62 v66.55,20.52 | v64.41,7.92 64.5,7.84 U506.6 64.5,6.32 65.13,5.69 U504.7 | X503.9 55.13,1.46 55.07,1.52 55.07,10.26 v54.76,10.57 | U502.4 58.02,9.64 57.4,10.26 57.4,10.46 57.81,10.87 v57.91,10.87
  Horizontal 0.152: v42.27,10.87 42.37,10.97 43.18,10.97 43.59,10.57 v54.76,10.57 56.39,10.57 56.69,10.87 v57.91,10.87 59.33,10.87 62.08,8.13 62.89,8.13 63.2,8.43 63.91,8.43 v64.41,7.92
  Vertical 0.152: v66.55,20.52 66.04,20.02 66.04,18.69 63.91,16.56 v63.91,15.44 63.91,8.43 v64.41,7.92
SPI_INT_MOSI  (via drill 0.15, 0.2)
  Top 0.152: v42.88,10.46 42.88,11 U101.32 | U505.24 67.73,21 v67.87,21.13 | v65.63,7.92 65.75,7.81 U506.7 65.73,6.91 65.73,5.89 65.63,5.78 U504.6 | 64.52,14.83 64.5,14.81 U501.3 64.52,14.72 v64.52,15.44 | X503.8 55.63,1.47 55.58,1.52 v55.58,9.86 | U502.3 58.52,10.06 58.32,10.26 v58.01,10.26
  Horizontal 0.152: v42.88,10.46 43.18,10.16 54.46,10.16 54.76,9.86 v55.58,9.86 57.61,9.86 v58.01,10.26 59.33,10.26 61.98,7.72 62.89,7.72 63.09,7.52 63.09,6.71 63.3,6.5 65.33,6.5 65.63,6.81 v65.63,7.92
  Vertical 0.152: v67.87,21.13 67.67,21.13 67.06,20.52 67.06,20.32 66.75,20.02 66.55,20.02 66.34,19.81 66.34,18.49 64.52,16.66 v64.52,15.44 64.52,9.04 v65.63,7.92
SPI_INT_SCK  (via drill 0.15, 0.2)
  Top 0.152: U101.30 42.47,9.99 v42.47,9.96 | U505.23 66.99,20.05 66.85,19.91 v66.85,19.3 | v66.65,7.92 67,7.57 U506.8 67,6.15 67.26,5.89 67.26,4.57 67.05,4.36 U504.4 | v65.23,15.54 65.23,14.78 U501.2 | X503.10 54.63,1.6 54.66,1.63 54.66,9.25 v54.56,9.35 | U502.2 v59.02,8.75 v59.03,8.74
  Horizontal 0.152: v42.47,9.96 42.77,9.65 53.75,9.65 54.05,9.35 v54.56,9.35 58.42,9.35 v59.03,8.74 60.45,8.74 62.99,6.2 66.24,6.2 66.65,6.6 v66.65,7.92
  Vertical 0.152: v66.85,19.3 66.65,19.1 66.65,18.29 65.23,16.87 v65.23,15.54 65.23,9.35 v66.65,7.92
VBAT  (via drill 0.2, 0.3)
  Top 0.152: U101.6 29.19,15.85 28.35,15.85 v27.23,16.97 | v21.74,18.9 21.57,18.9 U801.1 | v22.76,29.06 23.47,29.06 24.01,29.06 B601.1 v24.08,29.06 v25.3,29.06
  Top 0.254: R608.P$1 23.56,29.15 23.47,29.06
  Horizontal 0.152: v27.23,16.97 26.11,16.97 24.18,18.9 v21.74,18.9
  Vertical 0.152: v21.74,18.9 21.74,28.04 v22.76,29.06
VBUS  (via drill 0.2, 0.3)
  Top 0.15: R1112.P$1 v54.25,31.19
  Top 0.254: U302.5 43.89,32.51 44.91,32.51 | 44.91,32.51 44.91,30.38 42.77,28.25 42.77,28.02 U101.68 | 44.91,32.51 44.91,33.93 v45.21,34.24 | U1104.P$8 U1104.P$7 | v63.2,35.97 63.12,35.9 U1101.P$19
  Top 0.406: J301.VBUS 44.78,35.28 v45.21,34.85 | VBUS.P$1 46.23,34.34 46.13,34.44 45.41,34.44 v45.21,34.24
  Top 0.61: v45.21,34.85 v45.21,34.24
  Horizontal 0.254: v63.2,35.97 65.02,35.97 65.13,35.87
  Horizontal 1.016: v45.21,34.24 45.21,37.59 46.33,38.71 63.7,38.71 65.13,37.29 65.13,35.87 65.13,30.18
  Vertical 0.15: v58.42,32 58.42,31.5 58.12,31.19 v54.25,31.19
  Vertical 0.254: v58.42,32 59.23,32 v63.2,35.97
  Bottom 0.406: J302.1 43.44,36.62 v45.21,34.85
  other vias: 66.85,29.87 66.85,29.26 66.85,30.48
  pour Top (rank 2, no thermals): 66.75,29.16 67.87,29.16 68.17,28.85 68.17,28.14 68.28,28.04 69.9,28.04 69.9,29.06 69.8,29.16 68.48,29.16 67.97,29.67 67.97,30.38 67.77,30.58 66.75,30.58
  pour Horizontal (no thermals): 64.72,28.96 66.95,28.96 67.16,29.16 67.16,30.58 66.95,30.78 64.72,30.78
VDD_3V3_SENSORS  (via drill 0.2, 0.3)
  Top 0.15: C617.P$1 U603.8
  Top 0.152: U505.13 64.48,16.38 C514.P$1 C513.P$1 | 65.9,14.8 U501.1
  Top 0.25: 65.9,14.8 C513.P$1 | v62.18,10.36 C503.P$1 59.94,10.36 59.54,9.96 59.54,9.21 U502.1 59.89,8.82 U502.16
  Top 0.254: U501.16 U501.15 | U506.1 67,9.38 | U501.16 68.14,13.78 C502.P$1 | U501.1 65.8,14.63 66.65,14.63 | 66.65,14.63 66.65,13.78 U501.16 | v67.06,15.04 66.65,14.63 | U502.15 U502.16 | U504.1 67.14,2.86 v67.26,2.74 | X503.1 59.84,0.51 62.18,0.51 v63.5,1.83 64.01,2.34 64.63,2.34 U504.14 | C507.P$1 67.36,2.64 v67.26,2.74 | C506.P$1 67.33,2.68 v67.26,2.74
  Top 0.3: 59.2,16.66 C605.P$1
  Top 0.406: v62.59,20.73 59.84,20.73 59.2,20.08 C501.P$1 | U506.1 67.06,9.18 67.06,10.16 v67.26,10.36 68.07,10.36 68.18,10.47 C508.P$1
  Bottom 0.254: VDDA_3V1101.P$1 62.99,1.32 v63.5,1.83
  other vias: 68.38,14.43 67.87,14.43
  pour Power: 69.9,0 69.9,22.35 62.18,22.35 62.18,0
  pour Top (isolate 0.254, rank 3, no thermals): 60.15,18.69 60.15,15.75 59.64,15.24 58.62,15.24 58.01,14.63 57.3,14.63 57.2,14.73 57.2,18.69 57.4,18.9 59.94,18.9
  pour Top (isolate 0.254, no thermals): 66.65,15.44 69.6,15.44 69.7,15.34 69.7,13.51 69.6,13.41 65.23,13.41 64.82,13.82 64.82,16.26 65.23,16.66 66.14,16.66 66.45,16.36 66.45,15.65
VDD_3V3_SENSORS_EN  (via drill 0.2)
  Top 0.15: U603.5 57.85,13.37 58.01,13.21 58.01,12.39
  Top 0.152: U101.2 29.46,18.95 v29.46,19 | R635.P$2 R603.P$2 v55.47,11.79 57.41,11.79 58.01,12.39 | R620.P$2 54.66,19.91 v54.56,19.81
  Horizontal 0.152: v29.46,19 30.38,18.09 44.4,18.09 45.72,16.76 52.73,16.76 52.93,16.97 54.76,16.97 56.19,15.54 56.19,12.51 v55.47,11.79
  Vertical 0.152: v54.56,19.81 54.76,19.61 54.76,17.37 56.19,15.95 56.19,12.5 v55.47,11.79
VDD_3V3_SPEKTRUM  (via drill 0.3)
  Top 0.2: C1008.P$1 10.16,9.35
  Top 0.25: U1002.8 12.38,9.33 12.09,9.04 10.36,9.04 10.16,9.25 10.16,9.35 v10.16,10.06
  Top 0.254: D801.C 21.63,23.48 v20.73,24.38
  Power 0.406: v20.73,24.38 16.36,24.38 10.16,18.19 v10.16,10.06
  Bottom 0.406: J801.P$1 20.65,24.31 v20.73,24.38
VDD_3V3_SPEKTRUM_EN  (via drill 0.2)
  Top 0.152: U801.2 21.95,17.81 v21.95,16.66 | v15.24,10.06 R1002.P$2 14.37,9.54 U1002.5
  Horizontal 0.152: v16.56,14.02 16.87,14.33 19.61,14.33 v21.95,16.66
  Vertical 0.152: v15.24,10.06 15.24,12.7 v16.56,14.02
VDD_5V_BRICK  (via drill 0.2, 0.25)
  Top 0.152: U1101.P$21 62.12,37.13 62.48,37.49 | 62.48,37.49 v62.99,37.49 | 62.48,37.49 55.58,37.49 55.27,37.19 55.27,36.37 R1105.P$1
  Top 0.4: 68.92,37.29 C1101.P$1
  Bottom 0.152: VDD_5V_BRICK.P$1 v62.99,37.49
  other vias: 66.75,36.98 68.07,37.9 68.17,37.39
  pour Top (isolate 0.254, no thermals): 66.75,36.98 69.7,36.98 69.7,37.9 69.49,38.1 68.38,38.1 68.17,38.3 68.17,38.81 66.75,38.81
  pour Bottom (no thermals): 63.7,35.15 68.17,35.15 68.17,37.8 63.7,37.8
VDD_5V_HIPOWER
  Top 0.305: 36.78,37.59 U601.8
  Top 0.406: L201.P$1 36.78,37.59
  pour Top (isolate 0.254, rank 4, no thermals): 35.76,40.03 35.76,37.08 35.86,36.98 36.68,36.98 36.78,37.08 36.78,40.13 36.68,40.23 35.86,40.23 35.76,40.13
VDD_5V_IN  (via drill 0.2, 0.3)
  Top 0.15: RN1101.5 RN1101.6
  Top 0.152: RN1101.6 RN1101.7 55.94,27.79 55.58,27.43 55.58,25.91 54.97,25.3 VDD_5V_IN.P$1
  Top 0.25: VDD_5V_IN.P$1 54.66,25.2 54.66,22.25 54.25,21.84 v53.95,21.84 v52.73,21.84
  Top 0.254: U702.3 13.09,28.37 13.01,28.45 v13.01,29.46 13.01,30.04 L701.P$1 C702.P$1 | R609.P$2 v50.6,24.18 | 67.44,35.66 U1102.P$5 | 67.44,28.04 U1104.P$5 66.9,27.53 64.92,27.53 64.52,27.94 64.52,29.26 63.12,30.65 U1101.P$12 | U1102.P$6 67.44,36.37
  Top 0.406: L603.P$1 55.17,17.58 53.95,18.8 v53.95,21.84
  Top 0.61: v14.94,24.08 14.94,25.32 F1001.1
  Horizontal 0.406: v52.73,21.84 61.87,21.84 63.4,23.37
  Power 0.61: v35.76,36.47 33.43,36.47 32.92,36.98 32.72,36.98 31.5,38.2 17.68,38.2 13.01,33.53 v13.01,29.46 14.94,27.53 v14.94,24.08
  Bottom 0.254: U703.A3 U703.A2 | LED704.A LED701.A 10.87,36.03 10.87,33.12 13.01,30.99 v13.01,29.46
  Bottom 0.305: U703.A2 U703.A1
  other vias: 36.37,36.47 68.68,36.07 68.68,35.36 69.39,32.41 68.38,32.41 68.88,32.41 69.09,27.13 68.78,27.53 69.39,27.53 63.91,25.3 69.39,36.07 69.39,35.36 53.34,21.84
  pour Top (isolate 0.254, rank 3, no thermals): 67.26,36.47 69.8,36.47 69.8,22.66 62.69,22.66 62.69,25.7 67.26,25.7 67.26,28.85 68.17,28.85 68.17,31.6 67.26,31.6 67.26,33.12 68.17,33.12 68.17,35.36 67.26,35.36
  pour Power (no thermals): 34.75,36.68 63.6,36.68 63.6,35.15 69.9,35.15 69.9,40.44 34.75,40.44
  pour Bottom (no thermals): 50.8,20.83 47.14,20.83 47.14,26.01 50.8,26.01
  pour Bottom (no thermals): 51.31,20.83 51.31,26.01 51.92,26.01 51.92,20.83
  pour Bottom (no thermals): 52.43,20.83 52.43,26.01 56.18,26.01 56.18,20.83
  pour Top (no thermals): 35.66,36.58 35.66,35.36 36.98,35.36 36.98,36.58
  pour Horizontal (isolate 0.305, rank 6, no thermals): 64.92,40.03 69.6,40.03 69.9,39.73 69.9,22.66 69.6,22.35 63.3,22.45 62.99,22.76 62.99,26.01 63.3,26.31 64.31,26.31 64.62,26.62 64.62,39.73
  pour Top (isolate 0.254, no thermals): 52.32,22.45 55.17,22.45 55.17,20.73 52.32,20.73
VDD_5V_PERIPH  (via drill 0.2, 0.3)
  Top 0.25: L402.P$1 54.17,38.39 54.56,38 54.56,36.07 v54.25,35.76
  Top 0.406: v30.58,7.72 30.73,7.87 L203.P$1 | L404.P$1 v47.14,12.29 | v37.39,6.1 37.81,6.51 L403.P$1 | v61.37,1.22 L401.P$1 | v22.86,34.54 23.18,34.86 L202.P$1
  Power 0.61: v37.39,6.1 37.39,0.51 | 29.57,0.51 29.57,6.71 v30.58,7.72 | v47.14,12.29 47.14,0.51
  other vias: 61.37,25.1 60.76,25.1 61.16,23.06 61.77,23.06 61.47,22.56
  pour Power (no thermals): 61.67,0 61.67,36.27 22.56,36.27 22.56,34.24 43.08,34.24 43.08,31.19 59.13,31.19 59.13,0.81 28.85,0.81 28.85,0
  pour Top (no thermals): 61.77,25.81 61.77,24.89 60.55,24.89 60.55,25.81
  pour Top (isolate 0.254, no thermals): 60.55,24.18 62.59,24.18 63.4,24.99 64.41,24.99 64.52,24.89 64.52,22.05 64.41,21.95 60.55,21.95 60.45,22.05 60.45,24.08
VDD_5V_SENS  (via drill 0.2)
  Top 0.152: U101.29 40.03,11.72 v40.03,11.99 | R609.P$1 v52.22,23.37
  Top 0.25: R609.P$1 R610.P$1
  Horizontal 0.152: v52.22,23.37 45.52,23.37 43.99,24.89 42.27,24.89 41.66,24.28 v39.93,24.28
  Vertical 0.152: v40.03,11.99 39.12,12.9 39.12,23.47 v39.93,24.28
VDD_SERVO  (via drill 0.25, 0.3)
  Top 0.152: R1109.P$1 55.18,34.04 55.58,34.44 58.62,34.44 v58.73,34.54
  Top 0.254: D1.ANODE 9.21,20.46 9.65,20.02 10.27,20.02 R922.P$2 | U1103.P$7 U1103.P$8 | v62.69,36.47 62.62,36.41 U1101.P$20
  Top 0.406: v8.33,23.06 9.21,22.19 D1.ANODE | v51.21,39.93 51.71,39.93 VDD_SERVO.P$1
  Vertical 0.254: v58.73,34.54 60.76,34.54 v62.69,36.47
  other vias: 66.85,33.63 66.85,34.24 66.85,34.85
  pour Vertical (no thermals): 69.9,40.54 69.9,32.61 66.34,32.61 62.38,36.58 19.81,36.58 17.48,34.24 11.99,34.24 8.94,31.19 8.94,22.45 2.74,22.45 2.74,40.54
  pour Top (no thermals): 66.65,33.43 67.87,33.43 68.28,33.02 69.6,33.02 69.6,34.44 69.09,34.95 66.75,34.95
  pour Top (no thermals): 2.84,40.23 4.67,40.23 4.67,2.64 2.84,2.64
  pour Bottom (no thermals): 2.84,40.23 4.67,40.23 4.67,2.64 2.84,2.64
VDD_SERVO_IN  (via drill 0.3)
  Top 0.406: L901.P$2 11.37,24.19 v10.87,24.69 | v10.77,5.99 10.87,5.99 11.21,6.34 U1001.1
  Power 0.406: v10.87,24.69 11.38,24.18 11.38,21.44 7.82,17.88 7.82,6.4 8.23,5.99 v10.77,5.99
VDD_SERVO_SENS  (via drill 0.2)
  Top 0.152: R919.P$2 R918.P$1 13.61,21.23 13.61,20.42 v12.29,19.1 | U801.14 17.78,13.65 v17.78,13.72
  Horizontal 0.152: v17.78,13.72 17.48,13.41 15.65,13.41 14.94,14.12 v12.19,14.12
  Vertical 0.152: v12.19,14.12 12.7,14.63 12.7,18.69 v12.29,19.1

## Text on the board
tPlace: PX4FMU v2.4
bPlace: TLM | FMU PWR | FMU B/E | USB | SER2 | SER1 | Y | POWER | SPI | Z | X | SPKT | SWITCH | BUZZER | ADC | SER4 | DEBUG | PX4FMU 2.4 | (c) 2013 mjs/lm/jo | IO PWR | IO B/E | IO ACT | AIR | GPS | SER3 | CAN | I2C
Document: Optimized for good / manual soldering / accessibility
